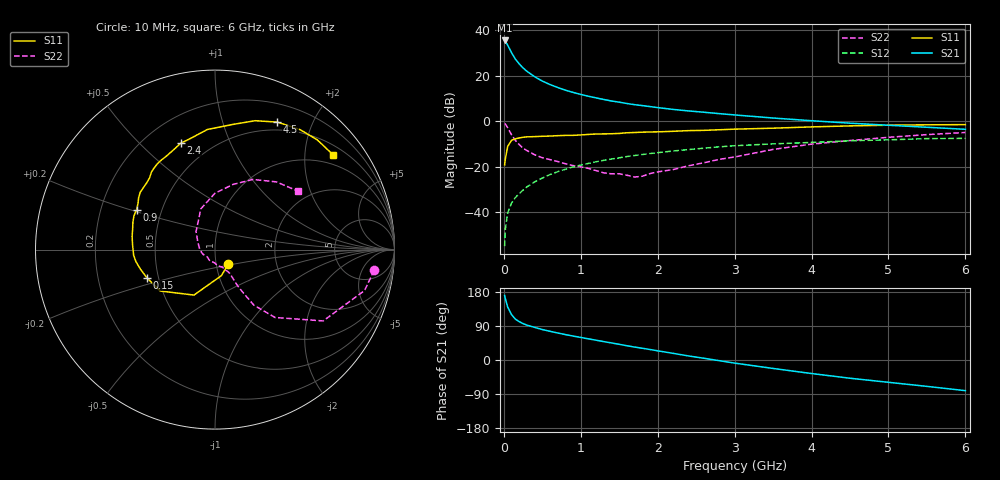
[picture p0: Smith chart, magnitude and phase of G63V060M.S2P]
! SIEMENS Small Signal Semiconductors
! BFG193
! Si NPN RF Bipolar Junction Transistor in SOT223
! VCE = 3 V  IC = 60 mA
! Common Emitter S-Parameters:  August  1996
# GHz  S  MA  R  50
!  f  S11  S21  S12  S22
! GHz  MAG  ANG  MAG  ANG  MAG  ANG  MAG  ANG
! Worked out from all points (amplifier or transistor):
!   36 points, 10 MHz to 6 GHz, reference 50 ohm
!   highest |S21| = 35.5 dB at 10 MHz (marker M1)
!   |S21| within 3 dB of that: start of sweep to 64.06 MHz
!   unconditionally stable (mu >= 1): 362 MHz to 2.4 GHz
!   at 250 MHz: K = 0.96, MSG = 26.8 dB, |S12| = -30.3 dB
!   at 1.4 GHz: K = 1.06, MAG = 11.3 dB, |S12| = -16.6 dB
!   at 6 GHz: K = 0.91, MSG = 2.0 dB, |S12| = -7.5 dB
!   S11 on the Smith chart (normalised r, x): 10 MHz: 1.14, -0.19; 150 MHz: 0.43, -0.16; 900 MHz: 0.36, +0.21; 2.4 GHz: 0.35, +0.67; 4.5 GHz: 0.40, +1.53; 6 GHz: 0.73, +2.66
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0.01  0.1095 -47.5  59.66 170.2  0.0018 90.0  0.8944 -7.4
0.02  0.1492 -76.1  57.02 161.8  0.0043 77.5  0.8639 -15.3
0.05  0.2792 -114.8  46.98 139.8  0.0097 70.1  0.7219 -33.4
0.1  0.383 -143.0  32.18 119.7  0.0159 69.4  0.505 -48.5
0.15  0.4114 -157.8  23.29 107.8  0.0211 67.7  0.3778 -55.0
0.2  0.4294 -165.3  18.25 101.2  0.0258 69.1  0.307 -56.4
0.25  0.4454 -171.3  14.83 96.1  0.0307 69.5  0.2559 -57.6
0.3  0.4542 -175.8  12.53 92.1  0.0361 70.2  0.227 -58.1
0.4  0.4598 177.0  9.526 86.1  0.0465 69.9  0.1837 -58.1
0.5  0.4676 170.9  7.634 80.4  0.0565 69.3  0.1581 -57.9
0.6  0.473 166.0  6.413 75.7  0.0674 68.1  0.1438 -59.4
0.7  0.4826 161.3  5.526 71.3  0.0779 66.7  0.1306 -62.3
0.9  0.4901 153.0  4.307 63.2  0.099 62.9  0.1063 -67.1
1.1  0.514 145.9  3.543 55.8  0.1186 59.2  0.0922 -79.4
1.3  0.5275 139.2  3.008 48.5  0.1388 55.1  0.0734 -91.9
1.6  0.5585 129.3  2.453 37.6  0.1679 48.1  0.0652 -122.1
2.2  0.6017 112.6  1.822 17.6  0.2223 34.3  0.0868 175.2
2.4  0.6228 107.9  1.687 10.7  0.239 29.9  0.1052 156.0
3.5  0.7048 81.8  1.178 -22.3  0.3189 2.6  0.2406 109.1
4.5  0.7909 63.9  0.907 -48.1  0.3722 -17.5  0.3769 74.5
5.5  0.8358 47.0  0.738 -69.6  0.416 -41.0  0.5093 47.8
6  0.8437 38.8  0.666 -80.9  0.4204 -54.4  0.5666 35.0
